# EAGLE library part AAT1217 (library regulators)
IC REG BST ADJ 0.75A SYNC TSOT23 Boost Switching Regulator IC Positive Adjustable 2.5V 1 Output 750mA (Switch) SOT-23-6 Thin, TSOT-23-6
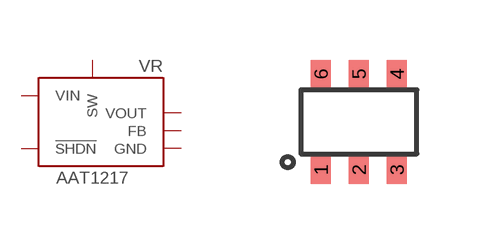
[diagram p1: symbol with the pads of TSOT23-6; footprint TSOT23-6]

Designator prefix VR

## AAT1217-1.2 (DIGIKEY: 863-1495-1-ND; MANUFACTURER: Skyworks Solutions Inc; MPN: AAT1217ICA-1.2-T1)  [TSOT23-6]
1  SW
2  GND
3  FB
4  !SHDN
5  VOUT
6  VIN

## Footprint TSOT23-6 (pad centres in mm)
TSOT23-6 drawn from http://www.skyworksinc.com/uploads/documents/AAT1217_202050B.pdf Digi-Key Part 863-1495-1-ND
smd 0.5 x 0.7: 1 -0.95,-1.2; 2 0,-1.2; 3 0.95,-1.2; 4 0.95,1.2; 5 0,1.2; 6 -0.95,1.2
